FUNCTION_BLOCK FB_Recipe
VAR_INPUT
	bRunOnCeDevice				: BOOL	:= TRUE;	(*在CE系统运行*)
	sgFilePath					: STRING(255)	:= 'Data\Recipe\';	(*文件路径*)
	eFileType					: E_FileType	:= eFileType_XML;	(*文件类型, 只支持 eFileType_XML 和 eFileType_BIN 两种类型*)
(*配方和备份(用来比较配方参数是否修改的)的类型必须一致, 把两个变量的首地址和数据长度传到功能块*)
	pRecData					: PVOID;			(*配方首地址*)
	pBakData					: PVOID;			(*配方备份数据首地址, 数据类型必须和配方一样*)
	nRecSize					: UDINT;			(*配方的字节数*)
	tAutoSaveRec				: TIME	:= T#10S;	(*配方改变后, 延时保存*)
END_VAR
VAR_OUTPUT
(*状态*)
	bInitialDone				: BOOL;	(*初始化完成*)
	bDone						: BOOL;
	bBusy						: BOOL;
	bError						: BOOL;
	nErrorId					: UDINT;
END_VAR
VAR
	i: INT;
(*Last status*)
	s_sLastExecuteResult		: ST_LastExecutionResult_File;
(*FB*)
	s_fbRecipeManager			: FB_RecipeManager_2;
	s_sRecipeData				: ST_RecipeData_2;
	s_sRecipeCtrl				: ST_RecipeCtrl_2;	(*配方相关的命令和状态*)
(*上载配方动作, 上载完成后, 不判断当前参数是否有改变*)
	s_ftRecipeLoad				: F_TRIG;
	s_tonLoadRecipe				: TON;
	s_bRecipeLoad				: BOOL;
(*参数改变, 延时触发写文件*)
	s_tonDataChange				: TON;
	s_bDataChange				: BOOL;
(*配方读写时间*)
	s_tActRecipeRead			: TIME;
	s_tActRecipeWrite			: TIME;
	s_tRecipeRead				: TIME;
	s_tRecipeWrite				: TIME;
	s_tonRecipeOperation		: TON;
	s_tonRecipeNotBusy			: TON;
END_VAR

(*
自定义错误代码
16#5F0A		数据缓冲区地址有误(备用)
16#5F0B		数据缓冲区字节数有误(备用)
*)

;
(*==================================================================
配置
==================================================================*)
	(*延时时间*)
	s_tonDataChange.PT					:= tAutoSaveRec;		(*参数修改后, 延时写入临时文件(作用是掉电保持)的时间*)
	s_tonLoadRecipe.PT					:= T#100MS;		(*上载配方时, 延时判断读取完成*)

	(*其他, 只针对TwinCAT PLC HMI, 第三方触摸屏的可以不设置*)
	s_sRecipeCtrl.i16DisplayFilesNum	:= 14;			(*Target Visualization中用到的'PH_RECIPE_FILE_NAME_DISPLAY'的数量, 如果是第三方HMI, 设置为0*)
	s_sRecipeCtrl.bRecipeNeedConfirm	:= TRUE;		(*上载, 保存, 删除是否需要确认. FALSE--不需要, TRUE--需要, 第三方触摸屏, 建议设置为FALSE*)	(*2020.10.10, 更改为FALSE*)
	s_sRecipeCtrl.bRecipeAutoRead		:= TRUE;		(*初始化时, 是否要从actRecipe中读取之前保存的参数*)
	s_sRecipeCtrl.bFileTypeDisplay		:= FALSE;		(*在'PH_RECIPE_FILE_NAME_DISPLAY'是否显示文件类型. FALSE--不显示, TRUE--显示*)
(*
	s_sRecipeCtrl.u16MaxTempFilesNum	:= 300;			(*保存300个临时文件*)
	s_sRecipeCtrl.u16KeepErrorFilesDay	:= 7;			(*错误文件保存7天*)
*)

(*==================================================================
变量地址是否有误
==================================================================*)
IF pRecData = 0 OR nRecSize <= 0 OR pBakData = 0 THEN
	bInitialDone := bBusy := bDone := FALSE;
	bError := TRUE;
	IF nRecSize > 0 THEN
		nErrorId := 16#5F0A;
	ELSE
		nErrorId := 16#5F0B;
	END_IF
	RETURN;
END_IF
(*变量的地址和长度*)
s_sRecipeData.stRecipeDataArr[1].pRecipeDataInfoADR			:= pRecData;
s_sRecipeData.stRecipeDataArr[1].u32RecipeDataInfoSIZEOF	:= nRecSize;
s_sRecipeData.stRecipeDataArr[1].sgRecipeDataInfoName		:= 'RecData';


(*==================================================================
判断参数是否变化, 变化后, 延时写入文件
==================================================================*)
s_tonRecipeNotBusy(IN := NOT s_sRecipeCtrl.sStatus.bBusy, PT := T#1S);
(*上载配方完成后, 把当前参数复制到临时参数中. 不写文件*)
s_ftRecipeLoad(CLK := s_sRecipeCtrl.sCmd.bRecipeLoad);
IF s_ftRecipeLoad.Q THEN
	s_tonLoadRecipe.IN := TRUE;
END_IF
s_tonLoadRecipe();
IF s_tonLoadRecipe.Q AND s_tonRecipeNotBusy.Q THEN
	s_bRecipeLoad := TRUE;
	s_tonLoadRecipe(IN := FALSE);
	s_tonDataChange(IN := FALSE);
END_IF

(*参数比较, 有变化时, 延时置位s_bDataChange, 将当前参数写到临时文件中*)
IF pRecData <> 0 AND nRecSize > 0 AND pBakData <> 0 THEN
	IF MEMCMP(pBakData, pRecData, nRecSize) <> 0 THEN
		s_tonDataChange(IN := FALSE);		(*重新计时*)
		s_tonDataChange(IN := s_sRecipeCtrl.sStatus.bInitialOk AND NOT s_bRecipeLoad);	(*上载配方后, 只复制参数, 不写入临时文件*)
		MEMCPY(pBakData, pRecData, nRecSize);	(*比较不同, 重新定时, 并把数据复制到局部变量*)
	END_IF
ELSE
	s_bRecipeLoad := FALSE;
END_IF

s_tonDataChange();
s_bDataChange := FALSE;
IF s_tonDataChange.Q AND s_tonRecipeNotBusy.Q THEN
	s_tonDataChange(IN := FALSE);
	s_bDataChange := TRUE;
END_IF

(*文件类型*)
IF eFileType = eFileType_BIN THEN
	s_fbRecipeManager.eFileType	:= eFileType_BIN;
ELSE
	s_fbRecipeManager.eFileType	:= eFileType_XML;
END_IF

(*==================================================================
调用配方程序, 根据实际情况修改文件夹路径: sgFolderName 和文件类型 eFileType
==================================================================*)
s_fbRecipeManager(
	sRecipeData				:= s_sRecipeData,		(*配方*)
	sgNetId					:= '',
	sgDeviceName			:= SEL(bRunOnCeDevice, 'C:\', '\Hard disk\'),		(*Device*)
	sgUsbDeviceName			:= SEL(bRunOnCeDevice, 'D:\', '\Hard disk2\'),		(*USB*)
	sgFolderName			:= sgFilePath,			(*文件夹, 支持多重, 写入时自动新建文件夹*)
	eFileType				:= ,					(*文件类型, 只支持 BIN 和 XML 两种类型*)
	bDataChange				:= s_bDataChange,		(*配方数据变更, 如果启用自动读取功能, 参数改变后, 会写到临时文件 actRecipe中, 掉电保持*)
	sRecipeCtrl				:= s_sRecipeCtrl);		(*和HMI的接口(按钮, 状态等)*)



(*记录读写时间*)
IF s_sRecipeCtrl.sStatus.bBusy THEN
	s_tonRecipeOperation(IN := TRUE, PT := T#1H);
	CASE s_fbRecipeManager.s_eOperateStep OF
		1..99:
			s_tActRecipeRead := s_tonRecipeOperation.ET;
		200..299:
			s_tActRecipeWrite := s_tonRecipeOperation.ET;
		300..399:
			s_tRecipeRead := s_tonRecipeOperation.ET;
		400..499:
			s_tRecipeWrite := s_tonRecipeOperation.ET;
	END_CASE
ELSE
	s_tonRecipeOperation(IN := FALSE);
END_IF

(*状态*)
bInitialDone	:= s_sRecipeCtrl.sStatus.bInitialOk;	(*初始化完成*)
bError			:= s_sRecipeCtrl.sStatus.bError;		(*报错*)
bBusy			:= s_sRecipeCtrl.sStatus.bBusy;
bDone			:= s_sRecipeCtrl.sStatus.bDone;
nErrorId		:= s_sRecipeCtrl.sStatus.u32ErrorId;
(*上一次触发的状态*)
MEMCPY(ADR(s_sLastExecuteResult), ADR(s_fbRecipeManager.s_sLastExecuteResult), SIZEOF(s_sLastExecuteResult));

END_FUNCTION_BLOCK
